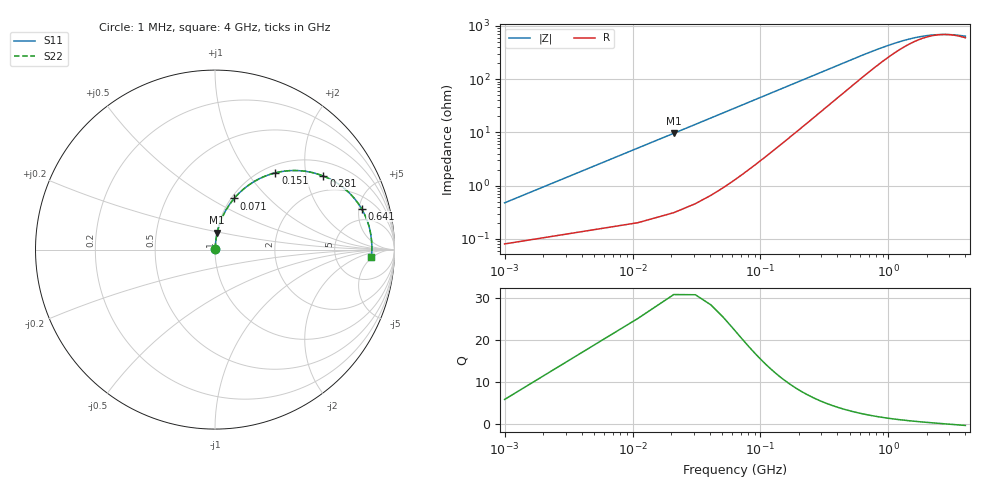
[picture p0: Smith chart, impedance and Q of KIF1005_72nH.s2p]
!version-2
!date-12.2020
!Series
# MHz S RI R 50
!Freq ReS11 ImS11 ReS21 ImS21 ReS12 ImS12 ReS22 ImS22
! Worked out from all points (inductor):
!   401 points, 1 MHz to 4 GHz, reference 50 ohm
!   read as one part in series: L = 72.7 nH near 21 MHz
!   highest Q = 25.2 at 21 MHz (marker M1), where L = 72.8 nH
!   self-resonance near 2.775 GHz
!   S11 on the Smith chart (normalised r, x): 1 MHz: 1.00, +0.01; 71 MHz: 1.03, +0.65; 151 MHz: 1.13, +1.37; 281 MHz: 1.44, +2.53; 641 MHz: 3.27, +5.31; 4 GHz: 13, -5
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1  0.000827 0.00468  0.9992 -0.00468  0.9992 -0.00468  0.000827 0.00468
11  0.00456 0.0504  0.9954 -0.0504  0.9954 -0.0504  0.00456 0.0504
21  0.0122 0.0947  0.9878 -0.0947  0.9878 -0.0947  0.0122 0.0947
31  0.024 0.1376  0.976 -0.1376  0.976 -0.1376  0.024 0.1376
41  0.0397 0.1785  0.9603 -0.1785  0.9603 -0.1785  0.0397 0.1785
51  0.059 0.2169  0.941 -0.2169  0.941 -0.2169  0.059 0.2169
71  0.1063 0.2847  0.8937 -0.2847  0.8937 -0.2847  0.1063 0.2847
101  0.1905 0.3614  0.8095 -0.3614  0.8095 -0.3614  0.1905 0.3614
151  0.3362 0.4277  0.6638 -0.4277  0.6638 -0.4277  0.3362 0.4277
211  0.4831 0.4387  0.5169 -0.4387  0.5169 -0.4387  0.4831 0.4387
281  0.6042 0.4096  0.3958 -0.4096  0.3958 -0.4096  0.6042 0.4096
351  0.6837 0.3681  0.3163 -0.3681  0.3163 -0.3681  0.6837 0.3681
431  0.7421 0.3217  0.2579 -0.3217  0.2579 -0.3217  0.7421 0.3217
641  0.8162 0.2286  0.1838 -0.2286  0.1838 -0.2286  0.8162 0.2286
671  0.822 0.2184  0.178 -0.2184  0.178 -0.2184  0.822 0.2184
981  0.8544 0.1424  0.1456 -0.1424  0.1456 -0.1424  0.8544 0.1424
1341  0.8668 0.0915  0.1332 -0.0915  0.1332 -0.0915  0.8668 0.0915
1651  0.8709 0.0626  0.1291 -0.0626  0.1291 -0.0626  0.8709 0.0626
2001  0.873 0.0382  0.127 -0.0382  0.127 -0.0382  0.873 0.0382
2671  0.8738 0.00437  0.1262 -0.00437  0.1262 -0.00437  0.8738 0.00437
3341  0.8728 -0.0212  0.1272 0.0212  0.1272 0.0212  0.8728 -0.0212
4000  0.871 -0.0424  0.129 0.0424  0.129 0.0424  0.871 -0.0424
